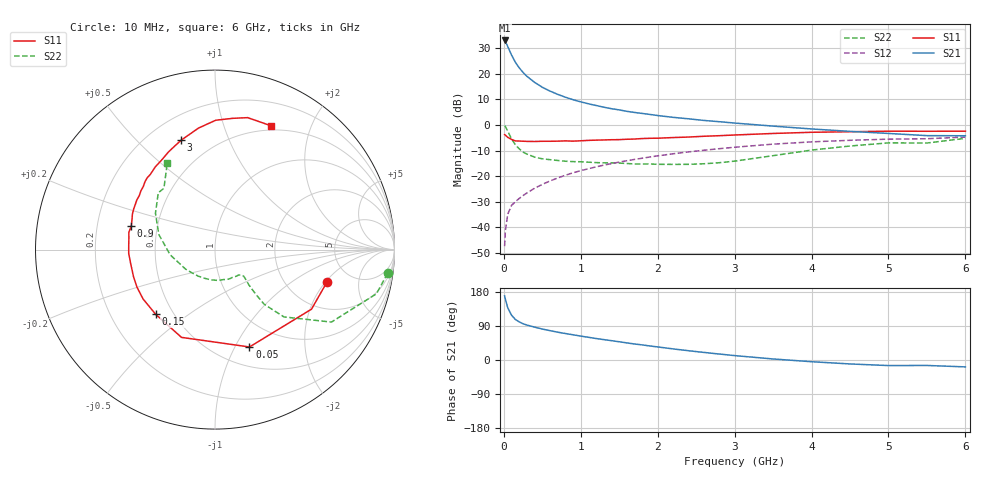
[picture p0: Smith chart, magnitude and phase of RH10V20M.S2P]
! SIEMENS Small Signal Semiconductors
! BFR106
! Si NPN RF Bipolar Junction Transistor in SOT23
! VCE = 10 V  IC = 20 mA
! Common Emitter S-Parameters:  August  1996
# GHz  S  MA  R  50
!  f  S11  S21  S12  S22
! GHz  MAG  ANG  MAG  ANG  MAG  ANG  MAG  ANG
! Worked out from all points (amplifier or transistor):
!   36 points, 10 MHz to 6 GHz, reference 50 ohm
!   highest |S21| = 33.0 dB at 10 MHz (marker M1)
!   |S21| within 3 dB of that: start of sweep to 60.15 MHz
!   unconditionally stable (mu >= 1): 389.2 MHz to 2.11 GHz
!   at 250 MHz: K = 0.87, MSG = 24.0 dB, |S12| = -27.6 dB
!   at 1.4 GHz: K = 1.07, MAG = 9.1 dB, |S12| = -15.1 dB
!   at 6 GHz: K = 0.98, MSG = 0.3 dB, |S12| = -4.7 dB
!   S11 on the Smith chart (normalised r, x): 10 MHz: 3.29, -2.08; 50 MHz: 0.71, -1.15; 150 MHz: 0.40, -0.38; 900 MHz: 0.35, +0.12; 3 GHz: 0.33, +0.68; 6 GHz: 0.45, +1.46
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0.01  0.6489 -16.4  44.8 169.1  0.0043 80.7  0.9707 -7.8
0.02  0.6318 -31.7  42.71 160.5  0.0086 72.7  0.9326 -15.3
0.05  0.5755 -70.5  34.32 138.3  0.018 63.6  0.7641 -31.9
0.1  0.5235 -110.9  23.26 118.3  0.0269 55.2  0.5371 -44.3
0.15  0.489 -132.6  16.77 107.0  0.0317 53.6  0.4106 -48.0
0.2  0.4861 -145.6  13.08 100.6  0.0368 55.8  0.3423 -47.6
0.25  0.4824 -154.4  10.61 95.6  0.0418 57.6  0.2958 -46.8
0.3  0.4786 -161.3  8.922 92.2  0.0471 60.4  0.2709 -46.1
0.4  0.4762 -170.2  6.799 86.7  0.0582 62.8  0.2362 -44.0
0.5  0.4812 -177.5  5.465 81.7  0.0692 64.9  0.2187 -42.8
0.6  0.4812 177.1  4.598 77.5  0.0808 66.0  0.2103 -43.4
0.7  0.4839 172.6  3.968 73.4  0.0922 66.6  0.2028 -44.7
0.9  0.4842 164.4  3.117 66.5  0.1166 66.5  0.1927 -47.2
1.1  0.5007 156.8  2.595 59.9  0.1399 65.5  0.1878 -53.1
1.3  0.5103 150.5  2.226 53.8  0.1645 64.1  0.1824 -58.8
1.6  0.527 141.6  1.849 45.1  0.2007 61.2  0.1772 -70.1
2.2  0.5684 125.8  1.411 29.3  0.274 54.5  0.1702 -98.3
3  0.6381 107.2  1.092 11.6  0.3679 43.6  0.1969 -146.6
3.5  0.6834 97.7  0.951 2.7  0.4229 36.3  0.2516 -173.4
4.5  0.738 82.3  0.751 -10.4  0.5025 20.5  0.3887 148.6
5.5  0.7544 69.7  0.62 -14.4  0.5395 9.3  0.4446 129.8
6  0.7573 65.5  0.616 -18.2  0.581 1.7  0.5488 119.0
